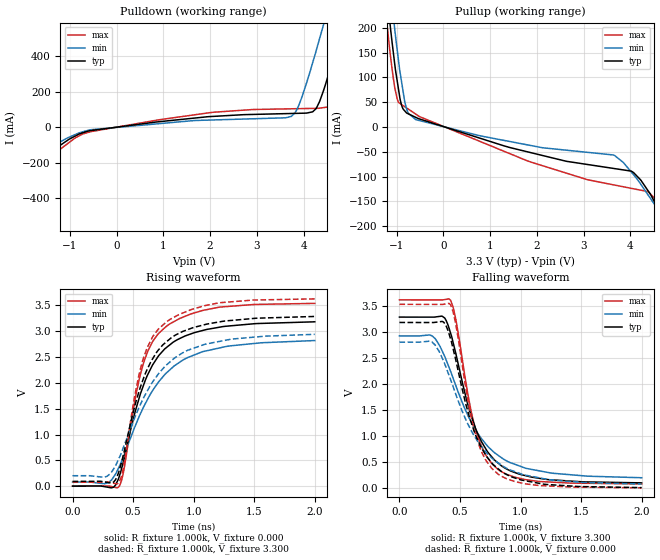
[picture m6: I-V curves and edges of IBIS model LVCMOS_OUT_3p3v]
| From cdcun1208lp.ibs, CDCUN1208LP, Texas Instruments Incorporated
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[Model]   LVCMOS_OUT_3p3v
Model_type   Output
Polarity   Non-Inverting
Enable   Active-High
Vmeas = 1.65
Vref = 1.65
Cref = 0pF
Rref = 50
|   typ   min   max
C_comp   6.1391pF   5.9693pF   6.2823pF
[Voltage Range]   3.3   2.97   3.63
[Temperature Range]   27   105   -40
[Pullup Reference]   3.3   2.97   3.63
[Pulldown Reference]   -0   0   0
[Power Clamp Reference]   3.3   2.97   3.63
[GND Clamp Reference]   0   0   0
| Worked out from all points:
|   slope of the pulldown table from 0 to 0.495 V, typ, clamps not added: 29 ohm
|   slope of the pullup table from 0 to 0.495 V, typ, clamps not added: 33.3 ohm
|   falling waveform, R_fixture 1.000k, V_fixture 3.300: 20-80 % time 258ps typ, 355ps min, 192ps max; typ from 3.29 V to 0.108 V
|   rising waveform, R_fixture 1.000k, V_fixture 0.000: 20-80 % time 282ps typ, 383ps min, 219ps max; typ from 0.007 V to 3.17 V
|   rising waveform, R_fixture 1.000k, V_fixture 3.300: 20-80 % time 281ps typ, 378ps min, 219ps max; typ from 0.097 V to 3.27 V
|   falling waveform, R_fixture 1.000k, V_fixture 0.000: 20-80 % time 254ps typ, 347ps min, 188ps max; typ from 3.19 V to 0.017 V
[Pulldown]
|   Voltage   I(typ)   I(min)   I(max)
-3.3V     -1.553A    -1.436A    -1.661A
-2.542V   -816.4mA   -708.9mA   -921.9mA
-2.263V   -557.1mA   -451mA     -650.6mA
-2.148V   -450.5mA   -352mA     -542.6mA
-1.77V    -205.4mA   -165.8mA   -251.3mA
-799.7mV  -39.35mA   -32.53mA   -49.54mA
3.738V    76.42mA    59.9mA     102.8mA
4.269V    103.7mA    428.3mA    105.5mA
4.619V    369.7mA    755.1mA    116.8mA
4.837V    572.8mA    966.7mA    217.9mA
5.306V    1.025A     1.42A      647mA
6.59V     2.284A     2.681A     1.903A
[Pullup]
|   Voltage   I(typ)   I(min)   I(max)
-3.3V     2.293A     2.365A     2.238A
-1.267V   320.9mA    395.1mA    260.9mA
-1.149V   214.6mA    289.3mA    156.2mA
-1.072V   150.3mA    223.2mA    98.45mA
-893.1mV  43.67mA    89.94mA    45.28mA
-778.6mV  27.91mA    34.05mA    37.99mA
-589mV    19.45mA    14.93mA    25.92mA
3.642V    -83.43mA   -56.32mA   -116.5mA
4.048V    -90.52mA   -93.86mA   -124.1mA
4.393V    -130.5mA   -138.8mA   -131.4mA
4.867V    -212.2mA   -211.5mA   -202.9mA
6.59V     -1.544A    -1.749A    -1.328A
[Ramp]
R_load = 1000
|   typ   min   max
dV/dt_r   1.89954/2.81989e-010   1.67848/3.80198e-010   2.1131/2.1855e-010
dV/dt_f   1.91052/2.57163e-010   1.69554/3.54129e-010   2.12161/1.90433e-010
[Falling Waveform]
R_fixture = 1.000k
V_fixture = 3.300
V_fixture_min = 2.970
V_fixture_max = 3.630
C_fixture = 0.000
|  time   V(typ)   V(min)   V(max)
0s        3.292V     2.931V     3.623V
270.4ps   3.291V     2.931V     3.622V
373.9ps   3.274V     2.537V     3.628V
422.4ps   2.984V     2.25V      3.616V
466.7ps   2.582V     1.97V      3.234V
563.9ps   1.623V     1.411V     1.825V
629ps     1.151V     1.124V     1.136V
813.1ps   492.3mV    640mV      367.9mV
1.213ns   174.6mV    313.8mV    127.3mV
2ns       107.9mV    206.5mV    87.14mV
[Rising Waveform]
R_fixture = 1.000k
V_fixture = 0.000
V_fixture_min = 0.000
V_fixture_max = 0.000
C_fixture = 0.000
|  time   V(typ)   V(min)   V(max)
0s        6.583mV    84.47mV    5.659mV
293.7ps   -16.42mV   70.82mV    8.469mV
387.9ps   209.1mV    394.7mV    11.31mV
421.4ps   495.2mV    583.1mV    285.2mV
514.7ps   1.422V     1.149V     1.655V
581.1ps   1.919V     1.505V     2.338V
666.8ps   2.362V     1.869V     2.813V
773.2ps   2.672V     2.183V     3.083V
1.073ns   3.004V     2.597V     3.39V
2ns       3.172V     2.811V     3.527V
[Rising Waveform]
R_fixture = 1.000k
V_fixture = 3.300
V_fixture_min = 2.970
V_fixture_max = 3.630
C_fixture = 0.000
|  time   V(typ)   V(min)   V(max)
0s        97.07mV    206.5mV    80.11mV
284.8ps   78.2mV     195.7mV    82.83mV
385.9ps   313.7mV    554.2mV    83.69mV
418.9ps   602.7mV    746.3mV    351mV
509.8ps   1.512V     1.303V     1.702V
577ps     2.025V     1.661V     2.407V
659.8ps   2.455V     2.008V     2.878V
773.2ps   2.783V     2.336V     3.167V
1.095ns   3.12V      2.741V     3.485V
2ns       3.275V     2.931V     3.614V
[Falling Waveform]
R_fixture = 1.000k
V_fixture = 0.000
V_fixture_min = 0.000
V_fixture_max = 0.000
C_fixture = 0.000
|  time   V(typ)   V(min)   V(max)
0s        3.189V     2.811V     3.537V
268.9ps   3.188V     2.812V     3.536V
362.9ps   3.198V     2.457V     3.537V
422.4ps   2.874V     2.092V     3.53V
465.9ps   2.461V     1.808V     3.149V
625.6ps   1.046V     978.6mV    1.059V
708.6ps   657.6mV    717mV      563.7mV
813.1ps   383.1mV    494.3mV    278.9mV
1.19ns    83.38mV    188.9mV    52.48mV
2ns       16.5mV     84.47mV    12.37mV
